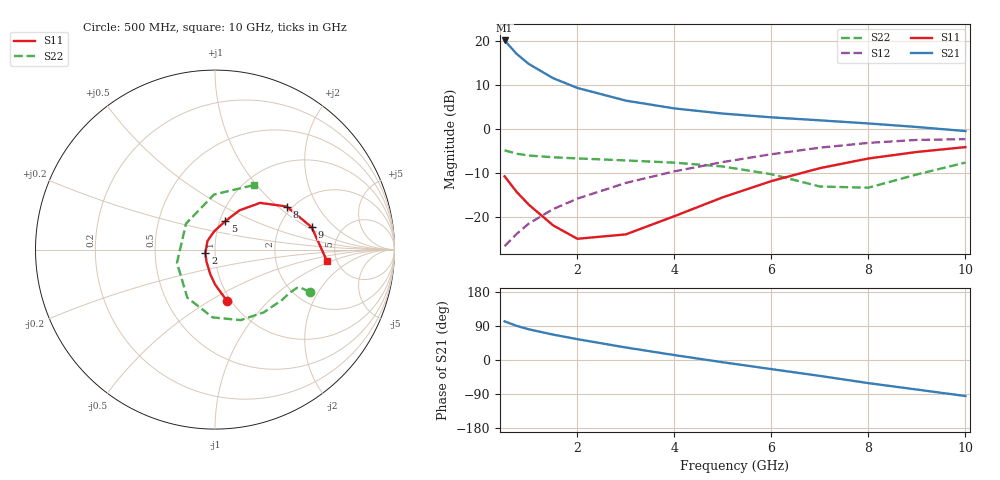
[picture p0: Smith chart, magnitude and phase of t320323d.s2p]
!AT-32032
!S-PARAMETERS at Vce=2.7V  Ic=10mA.  LAST UPDATED 05-29-98
# ghz s ma r 50
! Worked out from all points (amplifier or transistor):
!   13 points, 500 MHz to 10 GHz, reference 50 ohm
!   highest |S21| = 20.2 dB at 500 MHz (marker M1)
!   |S21| within 3 dB of that: start of sweep to 743.8 MHz
!   unconditionally stable (mu >= 1): 943.9 MHz to 3.002 GHz
!   at 1 GHz: K = 1.01, MAG = 17.6 dB, |S12| = -21.4 dB
!   at 4 GHz: K = 0.96, MSG = 7.2 dB, |S12| = -9.6 dB
!   at 10 GHz: K = 0.91, MSG = 0.9 dB, |S12| = -2.2 dB
!   lowest NFmin = 1.10 dB at 900 MHz
!   S11 on the Smith chart (normalised r, x): 500 MHz: 0.96, -0.60; 2 GHz: 0.90, -0.03; 5 GHz: 1.06, +0.35; 8 GHz: 1.87, +1.15; 9 GHz: 3.04, +1.09; 10 GHz: 4.17, -0.90
0.5  0.292 -77.0  10.23 102.0  0.047 68.0  0.577 -24.0
0.75  0.194 -90.0  7.179 90.0  0.065 68.0  0.528 -24.0
1  0.139 -101.0  5.527 81.0  0.085 68.0  0.504 -25.0
1.5  0.081 -126.0  3.813 67.0  0.124 64.0  0.481 -30.0
2  0.057 -161.0  2.954 55.0  0.163 59.0  0.467 -37.0
3  0.064 131.0  2.119 33.0  0.246 48.0  0.443 -52.0
4  0.103 92.0  1.728 13.0  0.333 35.0  0.418 -70.0
5  0.169 70.0  1.51 -6.0  0.425 21.0  0.378 -92.0
6  0.258 58.0  1.368 -24.0  0.521 6.0  0.309 -120.0
7  0.362 46.0  1.265 -42.0  0.619 -11.0  0.224 -161.0
8  0.466 31.0  1.166 -61.0  0.701 -30.0  0.217 138.0
9  0.553 13.0  1.063 -78.0  0.758 -50.0  0.307 91.0
10  0.628 -6.0  0.955 -95.0  0.773 -70.0  0.419 59.0
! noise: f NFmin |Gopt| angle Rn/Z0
0.9  1.1  0.15  87  0.15
1.8  1.3  0.23  159  0.11
2  1.4  0.26  173  0.11
2.5  1.5  0.32  -156  0.11
3  1.7  0.38  -128  0.17
3.5  1.9  0.45  -105  0.3
4  2  0.52  -84  0.5
